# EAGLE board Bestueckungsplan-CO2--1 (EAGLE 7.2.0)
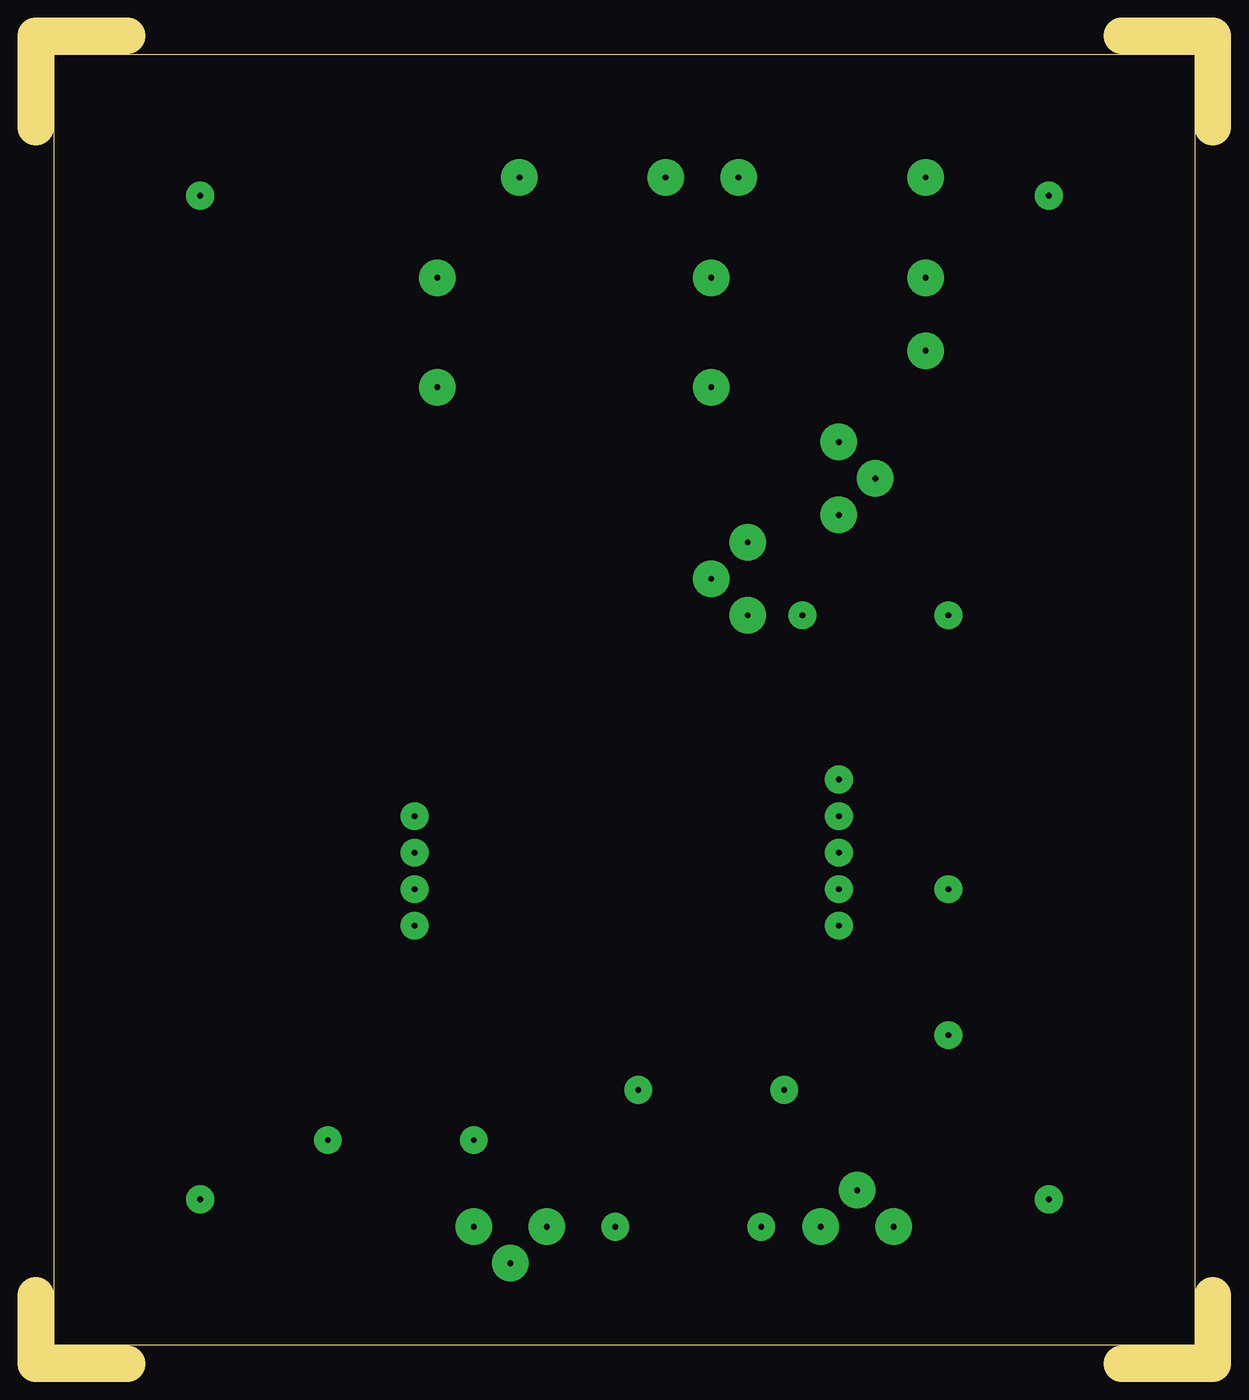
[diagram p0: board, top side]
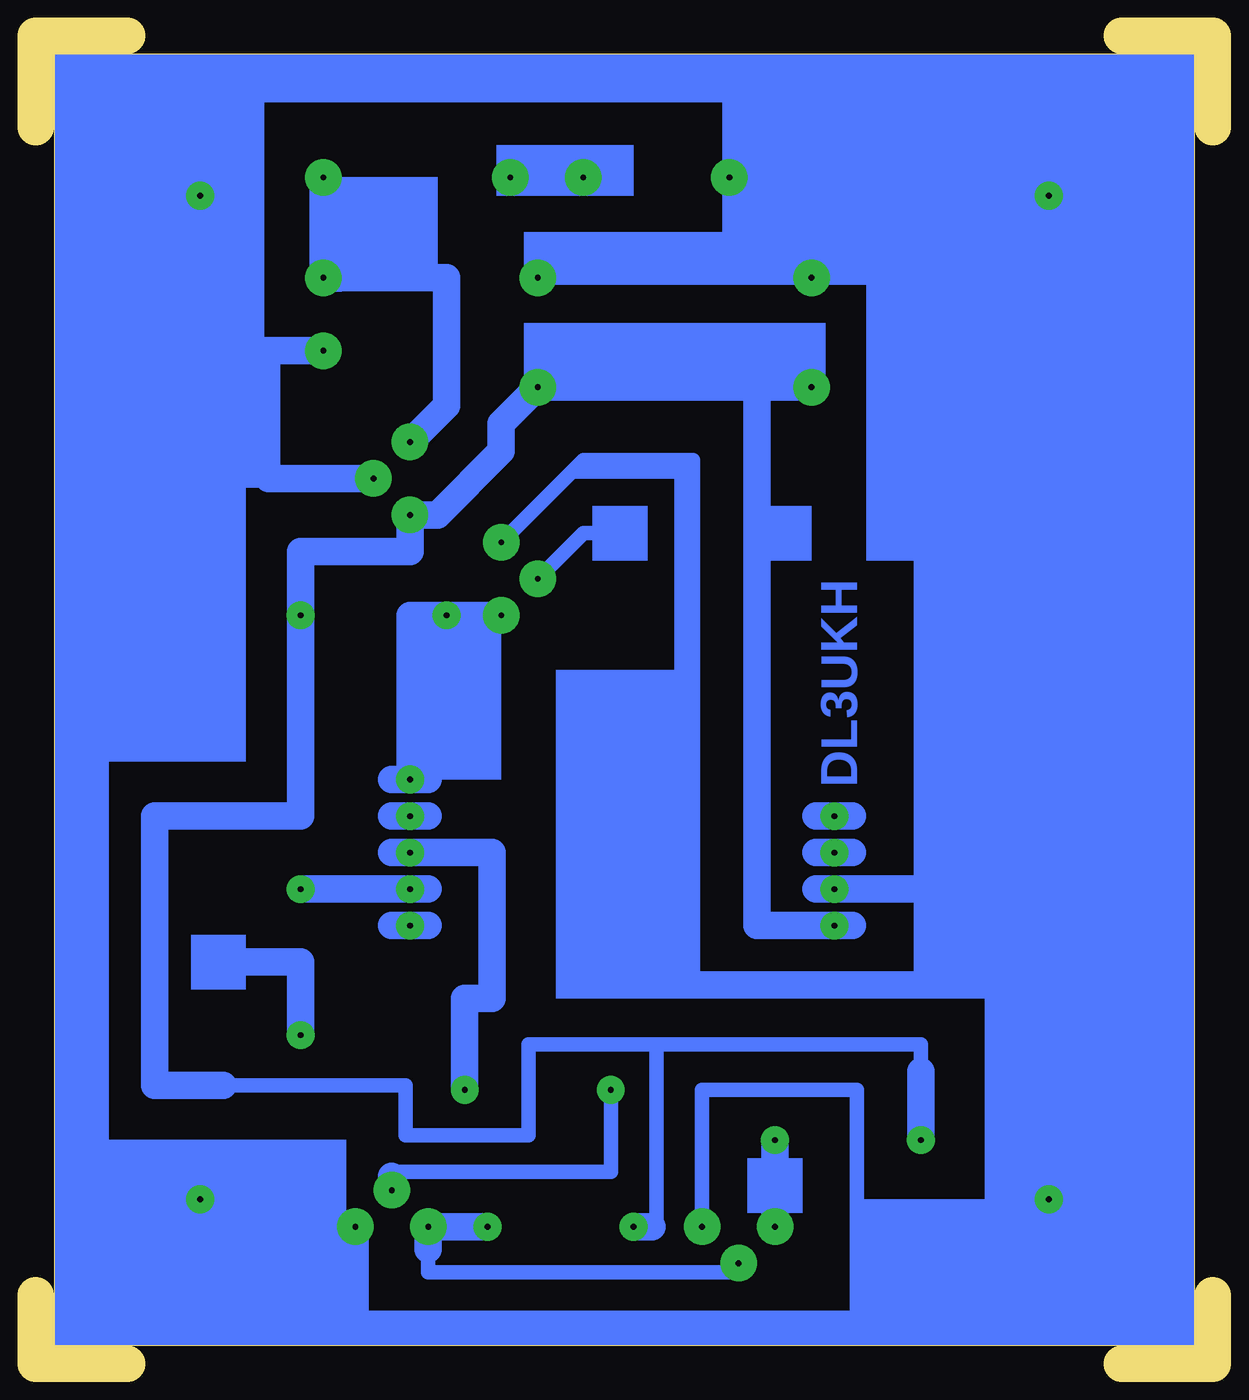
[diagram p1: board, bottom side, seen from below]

Size 81.91 x 92.39 mm. Coordinates in mm from the lower left corner, seen from the top.
Outline: 81.91,86.04 81.91,92.39 75.56,92.39
Outline: 81.91,4.76 81.91,0 75.56,0
Outline: 6.35,0 0,0 0,4.76
Outline: 0,86.04 0,92.39 6.35,92.39
Outline: 80.64,91.12 80.64,1.27 1.27,1.27 1.27,91.12 80.64,91.12
Copper layers (1*16): Top 0.035mm / dielectric 1.5mm / Bottom 0.035mm
Design rules "default": minimum track width 10mil, minimum drill 24mil, track to track 8mil, track to pad 8mil, pad to pad 8mil, via to via 8mil, smd to smd 8mil, copper to edge 40mil, drill to drill 8mil, minimum pad ring 10mil, minimum via ring 8mil, stop-mask expansion 4mil, vias tented up to drill 0mil, thermal gap 10mil

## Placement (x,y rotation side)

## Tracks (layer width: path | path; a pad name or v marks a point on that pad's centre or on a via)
S$1  (via drill 0.4 pad 1.93)
  Bottom 1.016: 52.07,23.18 52.07,23.81 | 55.88,35.56 56.2,35.56
  Bottom 1.93: 55.88,35.56 50.17,35.56 50.17,25.4 52.07,25.4 52.07,24.77 52.07,23.81 52.07,23.18 52.07,21.27 v52.07,19.05
S$2  (via drill 0.4 pad 1.93, 0.4 pad 2.54)
  Bottom 1.016: 68.9,19.37 56.2,19.37 56.2,15.88 47.62,15.88 47.62,22.22 38.74,22.22 | 39.05,9.53 38.74,9.53 38.74,22.22 | 38.74,22.22 20.32,22.22 20.32,20.32 | 63.5,56.52 v63.5,52.07 63.5,38.1
  Bottom 1.93: v27.94,67.94 31.75,67.94 | 31.75,67.94 v46.99,67.94 49.53,65.41 49.53,63.5 53.98,59.05 v55.88,59.05 55.88,56.52 63.5,56.52 63.5,38.1 73.66,38.1 73.66,19.37 68.9,19.37 | v26.35,30.48 31.75,30.48 31.75,67.94 | v20.32,15.56 20.32,20.32 | v40.32,9.53 39.05,9.53
S$3  (via drill 0.4 pad 2.54)
  Bottom 1.93: v43.82,82.55 v48.9,82.55
S$4  (via drill 0.4 pad 1.93)
  other vias: 55.88,38.1
S$5  (via drill 0.4 pad 2.54)
  Bottom 1.93: v61.91,82.55 v61.91,75.56 53.34,75.56 53.34,66.67 v55.88,64.14
S$6  (via drill 0.4 pad 1.93, 0.4 pad 2.54)
  Bottom 1.93: v30.48,15.56 v30.48,9.53
S$7  (via drill 0.4 pad 1.93)
  Bottom 1.93: v55.88,33.02 v63.5,33.02
S$8  (via drill 0.4 pad 1.93)
  other vias: 11.43,11.43
S$9  (via drill 0.4 pad 1.93)
  other vias: 11.43,81.28
S$10  (via drill 0.4 pad 1.93, 0.4 pad 2.54)
  Bottom 1.016: 20.32,33.02 20.32,26.04 | 20,33.02 12.7,33.02 12.7,75.56 20.32,75.56 | v61.91,70.48 65.41,70.48 | 65.41,70.48 65.41,61.6 58.74,61.6 v58.42,61.6 | 65.41,70.48 66.36,70.48 70.48,70.48 | 70.48,70.48 70.48,88.27 33.66,88.27 v33.66,82.55 33.66,75.56 | 33.66,75.56 v27.94,75.56 20.32,75.56 | 33.66,75.56 v46.99,75.56 | 70.48,70.48 78.42,70.48 78.42,3.17 59.69,3.17 | 59.69,3.17 59.69,3.49 | 59.69,3.17 24.77,3.17 24.77,19.05 35.56,19.05 v35.56,9.53 | 20.32,33.34 20.32,75.56
  Bottom 1.93: v26.35,33.02 20.32,33.02 20,33.02 | 58.74,61.6 65.72,61.6 | v61.91,70.48 66.36,70.48 | 59.69,3.49 v59.69,9.53 60.64,9.53
S$11  (via drill 0.4 pad 1.93)
  other vias: 55.88,30.48
S$12  (via drill 0.4 pad 1.93)
  Bottom 1.016: 67.94,27.94 69.85,27.94
  Bottom 1.93: v63.5,22.86 63.5,27.94 67.94,27.94
S$13
  Bottom 1.93: 25.08,38.1 27.62,38.1 | 25.08,35.56 27.62,35.56 | 54.61,38.1 57.15,38.1 | 54.61,40.64 57.15,40.64 | 54.61,30.48 57.15,30.48 | 54.61,33.02 57.15,33.02 | 25.08,33.02 27.62,33.02 | 54.61,35.56 57.15,35.56 | 25.08,30.48 27.62,30.48
S$14  (via drill 0.4 pad 1.93)
  other vias: 26.35,35.56
S$15  (via drill 0.4 pad 1.93)
  other vias: 26.35,38.1
S$16  (via drill 0.4 pad 1.93, 0.4 pad 2.54)
  Bottom 1.016: v33.02,6.98 33.66,6.35 54.61,6.35 54.61,7.94
  Bottom 1.93: v50.48,9.53 v54.61,9.53 54.61,7.94
S$17  (via drill 0.4 pad 1.93, 0.4 pad 2.54)
  Bottom 1.016: v49.53,52.07 v53.34,52.07 55.88,52.07
  Bottom 1.93: v49.53,52.07 55.88,52.07 v55.88,40.64
S$18  (via drill 0.4 pad 2.54)
  Bottom 1.016: v49.53,57.15 43.82,62.87 36.2,62.87 36.2,26.04
S$19  (via drill 0.4 pad 2.54)
  Bottom 1.016: v46.99,54.61 43.82,57.79 41.28,57.79
S$20  (via drill 0.4 pad 1.93, 0.4 pad 2.54)
  Bottom 1.016: 57.15,13.02 57.15,13.33 41.91,13.33 v41.91,19.05
  Bottom 1.93: v57.15,12.06 57.15,13.02
S$23  (via drill 0.4 pad 1.93)
  other vias: 55.88,35.56
S$29  (via drill 0.4 pad 1.93)
  other vias: 70.48,11.43
S$34  (via drill 0.4 pad 1.93)
  other vias: 70.48,81.28
(copper drawn outside any net)
  shapes: Bottom area x35

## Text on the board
Bottom: DL3UKH
Pads: AUF BESTÜCKUNGS-SEITE GESEHEN
Vias: 3 | 1 | 2 | 3 | 1 | 2
tOrigins: µA7805 | 2N7000 | 12 Volt | Kat | - | + | 1N4002 | Eing. | Ausg. | S | D | + | Masse | G | 470µ | 4700µ | 4700µ | BC547c | + | + | Eing. | 1N4002 | + | µA7805 | S | 5 Volt | - | 4,7K | 2N7000 | D | Katode | Anode | K | E | Kat | B | Für Anschlüsse | Sensor CO2 | Siehe Stromlaufplan | Auf Leiterzugseite anlöten | Auch die 5,0Volt | 4,7K | 75K | Leiterplatte: | 4,7K | 1,5mm dick | Cevausit | 2N7000 | B | S | 4,7K | E | Alles mit 0,8mm vorbohren ! | D | K | Aufbohren: | G | BC547c | 1N4002 1,0mm | µA7805 1,0mm | 4stck Befestigungs-Bohrungen 3,5mm | Sensor CO2 Anschlüsse 1,0mm | 2stck. Elkos 4700µ 1,0mm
